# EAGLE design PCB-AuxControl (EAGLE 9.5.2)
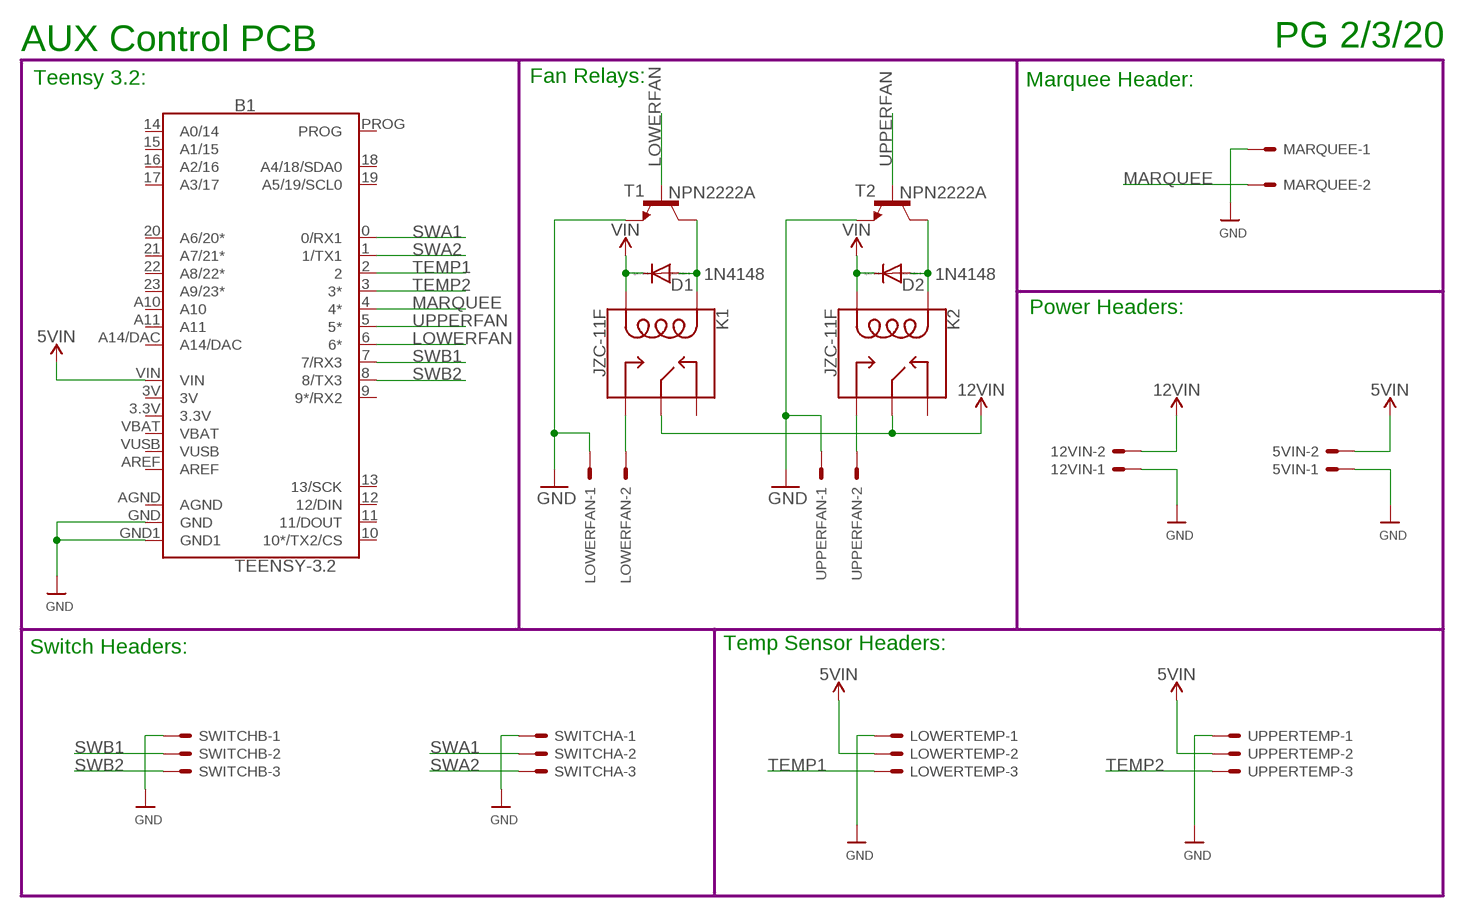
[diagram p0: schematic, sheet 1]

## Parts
5VIN  KK-156-2  [KK-156-2]
12VIN  KK-156-2  [KK-156-2]
B1  TEENSY-3.2  TEENSY-3.1SILK  [TEENSY-3.1]
D1  1N4148  1N4148DO35-7  [DO35-7]
D2  1N4148  1N4148DO35-7  [DO35-7]
K1  JZC-11F  RELAY-SPDT-JZC-11F  [RELAY-JZC]
K2  JZC-11F  RELAY-SPDT-JZC-11F  [RELAY-JZC]
LOWERFAN  KK-156-2  [KK-156-2]
LOWERTEMP  KK-156-3  [KK-156-3]
MARQUEE  KK-156-2  [KK-156-2]
SWITCHA  KK-156-3  [KK-156-3]
SWITCHB  KK-156-3  [KK-156-3]
T1  NPN2222A  BC337  [TO92]
T2  NPN2222A  BC337  [TO92]
UPPERFAN  KK-156-2  [KK-156-2]
UPPERTEMP  KK-156-3  [KK-156-3]

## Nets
5VIN: 5VIN.2 B1.VIN D1.C D2.C K1.1(COIL2) K2.1(COIL2) LOWERTEMP.2 UPPERTEMP.2 ; supply symbol labelled VIN
12VIN: 12VIN.2 K1.4(MAIN) K2.4(MAIN)
GND: 5VIN.1 12VIN.1 B1.GND B1.GND1 LOWERFAN.1 LOWERTEMP.1 MARQUEE.1 SWITCHA.1 SWITCHB.1 T1.1(E) T2.1(E) UPPERFAN.1 UPPERTEMP.1
LOWERFAN: B1.6(6*) T1.2(B)
MARQUEE: B1.4(4*) MARQUEE.2
N$3: K2.3(NO) UPPERFAN.2
N$4: K1.3(NO) LOWERFAN.2
RELAY1: D1.A K1.5(COIL1) T1.3(C)
RELAY2: D2.A K2.5(COIL1) T2.3(C)
SWA1: B1.0(0/RX1) SWITCHA.2
SWA2: B1.1(1/TX1) SWITCHA.3
SWB1: B1.7(7/RX3) SWITCHB.2
SWB2: B1.8(8/TX3) SWITCHB.3
TEMP1: B1.2 LOWERTEMP.3
TEMP2: B1.3(3*) UPPERTEMP.3
UPPERFAN: B1.5(5*) T2.2(B)
Unconnected: B1.9(9*/RX2) B1.10(10*/TX2/CS) B1.11(11/DOUT) B1.12(12/DIN) B1.13(13/SCK) B1.14(A0/14) B1.15(A1/15) B1.16(A2/16) B1.17(A3/17) B1.18(A4/18/SDA0) B1.19(A5/19/SCL0) B1.20(A6/20*) B1.21(A7/21*) B1.22(A8/22*) B1.23(A9/23*) B1.A10 B1.A11 B1.A14/DAC B1.AREF B1.PROG K1.2(NC) K2.2(NC)

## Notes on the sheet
- AUX Control PCB | PG 2/3/20
- Teensy 3.2: | Fan Relays: | Marquee Header:
- Power Headers:
- Switch Headers: | Temp Sensor Headers:

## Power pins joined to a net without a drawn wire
3.3V: B1.3.3V
3V: B1.3V
AGND: B1.AGND
VBAT: B1.VBAT
VUSB: B1.VUSB

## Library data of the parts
5VIN 12VIN LOWERFAN MARQUEE UPPERFAN = con-molex:KK-156-2: KK 156 HEADER; MF: MOLEX; OC_FARNELL: unknown; OC_NEWARK: unknown
B1 = SparkFun-Boards:TEENSY-3.1: Teensy 3+ Footprint Mechanical footprint with connectors for Teensy Development Board with ARM Cortex. SparkFun Products: Teensy 3.2 Teensy LC; SF_ID: DEV-12646
D1 D2 = diode:1N4148: DIODE
K1 K2 = SparkFun-Electromechanical:RELAY-SPDT: SPDT Electromechanical Relay Single-pole, double-throw sealed relays. When current is applied to the coil, it throws a simple changeover switch, terminating the connection from the NC contact to ground and closing the NO contact. Use them to switch high voltage/high current devices. SparkFun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; PROD_ID: COMP-09533; SF_SKU: COM-00100
LOWERTEMP SWITCHA SWITCHB UPPERTEMP = con-molex:KK-156-3: KK 156 HEADER Source: http://www.molex.com/pdm_docs/sd/026604100_sd.pdf; MF: MOLEX; OC_FARNELL: unknown; OC_NEWARK: unknown
T1 T2 = transistor:BC337: NPN TRANSISTOR

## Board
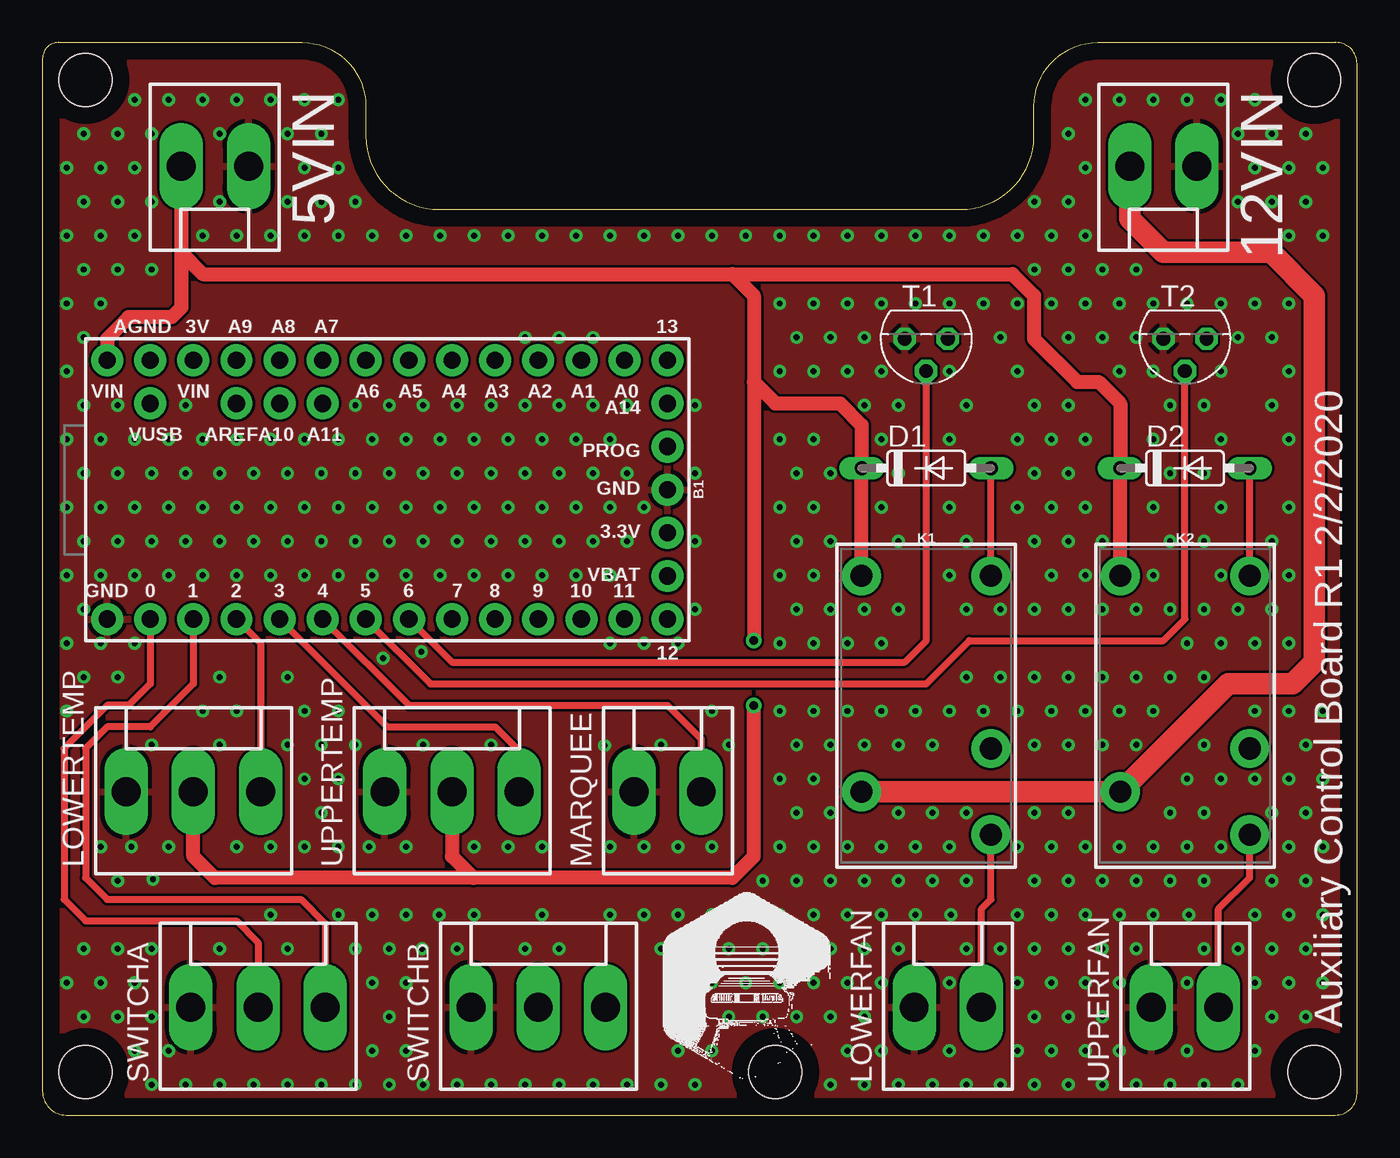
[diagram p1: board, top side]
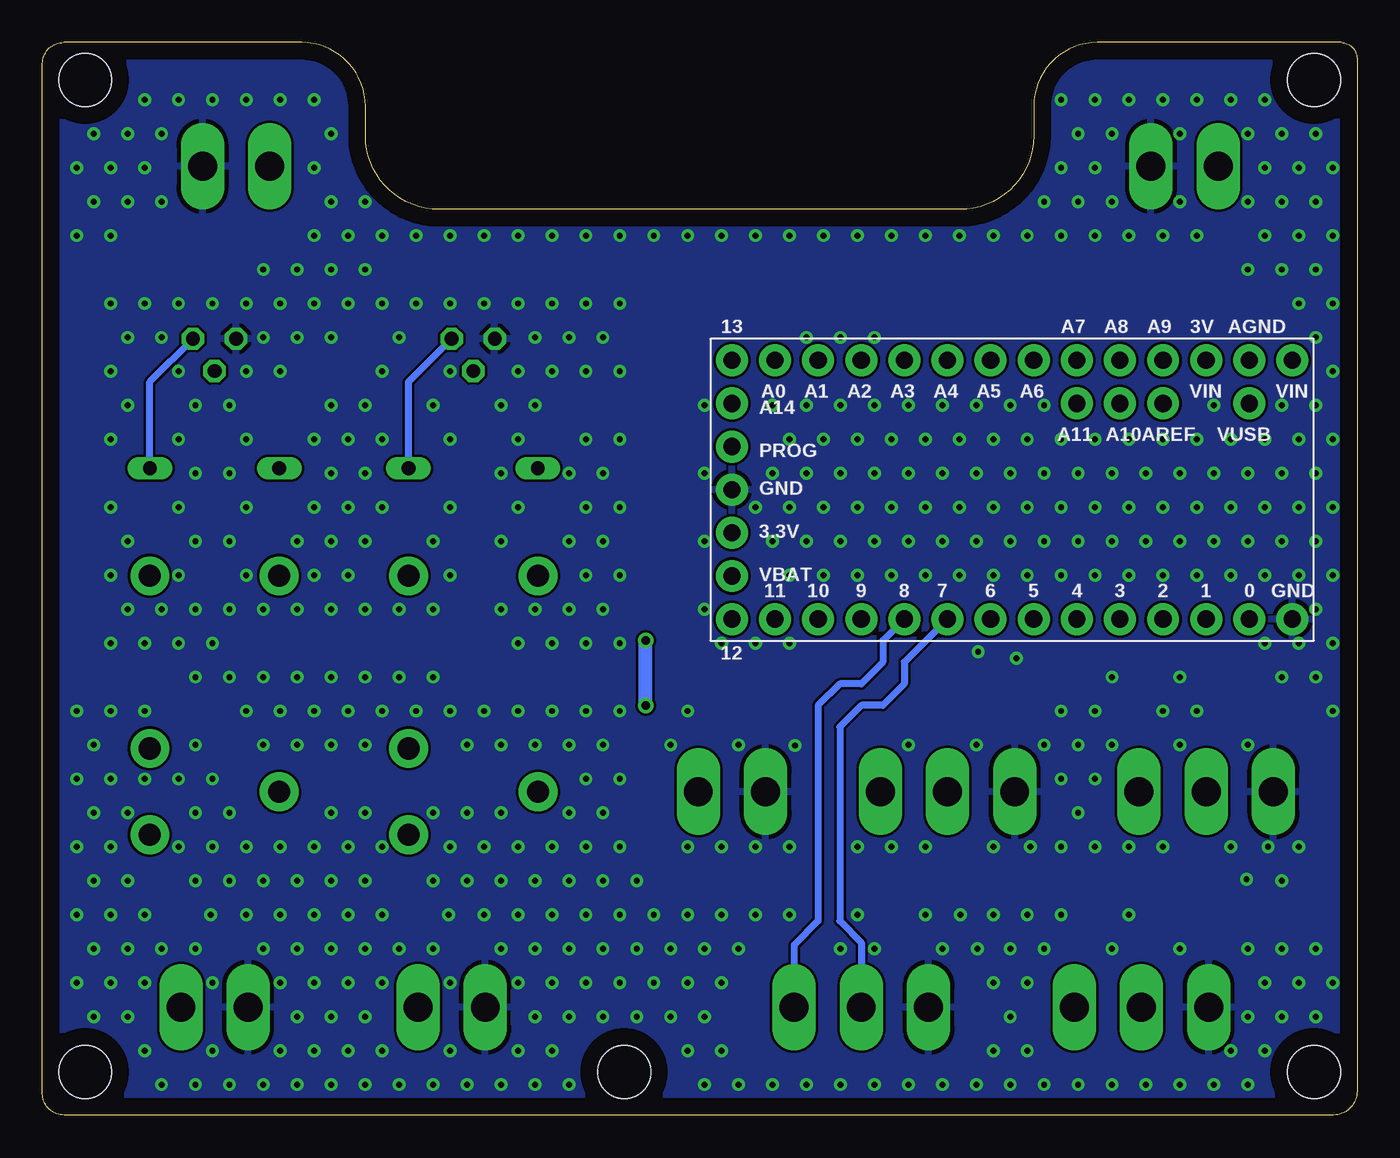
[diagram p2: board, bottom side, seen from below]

Size 77.45 x 63.17 mm. Coordinates in mm from the lower left corner, seen from the top.
Outline: 0,62.23 0,1.4 arc90 1.4,0 76.18,0 arc90 77.45,1.27 77.45,61.92 arc90 76.2,63.17 62.17,63.17 arc90 58.42,59.41 58.42,57.68 arc-90 54.08,53.34 23.39,53.34 arc-90 19.05,57.68 19.05,59.41 arc90 15.29,63.17 0.94,63.17 arc90 0,62.23
Copper layers (1*16): Top 0.035mm / dielectric 1.5mm / Bottom 0.035mm
Design rules "default": minimum track width 6mil, minimum drill 0.35mm, track to track 6mil, track to pad 6mil, pad to pad 6mil, via to via 6mil, smd to smd 6mil, copper to edge 40mil, drill to drill 6mil, minimum pad ring 10mil, minimum via ring 8mil, stop-mask expansion 4mil, vias tented up to drill 0.5mm, thermal gap 10mil
Holes 3.1 mm at 2.54,2.54 74.93,2.54 74.93,60.96 2.54,60.96 43.18,2.54

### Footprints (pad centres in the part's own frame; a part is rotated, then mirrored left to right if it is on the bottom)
KK-156-2 = drill 1.7 pad 2.184 long: 1 -1.98,0; 2 1.98,0
TEENSY-3.1 = drill 1.016 pad 1.88: 0 7.62,-13.97; 1 7.62,-11.43; 2 7.62,-8.89; 3 7.62,-6.35; 3.3V 2.54,16.51; 3V -7.62,-11.43; 4 7.62,-3.81; 5 7.62,-1.27; 6 7.62,1.27; 7 7.62,3.81; 8 7.62,6.35; 9 7.62,8.89; 10 7.62,11.43; 11 7.62,13.97; 12 7.62,16.51; 13 -7.62,16.51; 14 -7.62,13.97; 15 -7.62,11.43; 16 -7.62,8.89; 17 -7.62,6.35; 18 -7.62,3.81; 19 -7.62,1.27; 20 -7.62,-1.27; 21 -7.62,-3.81; 22 -7.62,-6.35; 23 -7.62,-8.89; A10 -5.08,-6.35; A11 -5.08,-3.81; A14/DAC -5.08,16.51; AGND -7.62,-13.97; AREF -5.08,-8.89; GND 0,16.51; GND1 7.62,-16.51; PROG -2.54,16.51; VBAT 5.08,16.51; VIN -7.62,-16.51; VUSB -5.08,-13.97
DO35-7 = drill 0.813 long: A 3.81,0; C -3.81,0
RELAY-JZC = drill 1.3 pad 2.286: 1 3.81,-8.89; 2 -3.81,1.27; 3 -3.81,6.35; 4 3.81,3.81; 5 -3.81,-8.89
KK-156-3 = drill 1.7 pad 2.184 long: 1 -3.96,0; 2 0,0; 3 3.96,0
TO92 = drill 0.813 octagon: 1 1.27,0; 2 0,1.905; 3 -1.27,0

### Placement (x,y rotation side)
5VIN  10.16,55.88 180 top
12VIN  66.04,55.88 180 top
B1  20.32,36.83 270 top
D1  52.07,38.1 0 top
D2  67.31,38.1 0 top
K1  52.07,22.86 180 top
K2  67.31,22.86 180 top
LOWERFAN  53.34,6.35 0 top
LOWERTEMP  8.89,19.05 0 top
MARQUEE  36.83,19.05 0 top
SWITCHA  12.7,6.35 0 top
SWITCHB  29.21,6.35 0 top
T1  52.07,45.72 180 top
T2  67.31,45.72 180 top
UPPERFAN  67.31,6.35 0 top
UPPERTEMP  24.13,19.05 0 top

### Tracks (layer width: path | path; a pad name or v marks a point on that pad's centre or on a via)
5VIN  (via drill 0.5)
  Top 0.813: K2.1 D2.C 63.5,41.91 62.23,43.18 60.96,43.18 58.42,45.72 58.42,48.26 57.15,49.53 40.64,49.53 | K1.1 D1.C 48.26,40.64 46.99,41.91 43.18,41.91 41.91,43.18 | 25.4,13.97 40.64,13.97 41.91,15.24 v41.91,24.13 | 25.4,13.97 10.16,13.97 8.89,15.24 LOWERTEMP.2 | 41.91,43.18 v41.91,27.94 | 40.64,49.53 41.91,48.26 41.91,43.18 | B1.VIN 3.81,45.72 5.08,46.99 7.62,46.99 8.18,47.55 8.18,50.8 | 5VIN.2 8.18,50.8 | 8.18,50.8 9.45,49.53 40.64,49.53 | UPPERTEMP.2 24.13,15.24 25.4,13.97
  Bottom 0.813: v41.91,24.13 v41.91,27.94
12VIN
  Top 1.27: K1.4 K2.4 69.85,25.4 73.66,25.4 74.93,26.67 74.93,48.26 72.39,50.8 66.04,50.8 64.06,52.78 12VIN.2
GND  (via drill 0.35)
  other vias: 2.44,5.8 1.44,7.8 2.44,9.8 1.44,23.8 2.44,25.8 1.44,27.8 2.44,29.8 1.44,31.8 2.44,33.8 1.44,35.8 2.44,37.8 1.44,39.8 2.44,41.8 1.44,43.8 2.44,45.8 1.44,47.8 2.44,49.8 1.44,51.8 2.44,53.8 1.44,55.8 2.44,57.8 4.44,5.8 3.44,7.8 4.44,9.8 4.44,13.8 3.44,15.8 4.44,25.8 3.44,27.8 3.44,31.8 4.44,33.8 3.44,35.8 4.44,37.8 3.44,39.8 4.44,41.8 3.44,47.8 4.44,49.8 3.44,51.8 4.44,53.8 3.44,55.8 4.44,57.8 6.44,1.8 5.44,3.8 6.44,5.8 5.44,7.8 6.44,9.8 6.44,21.8 5.44,27.8 5.44,31.8 6.44,33.8 5.44,35.8 6.44,37.8 5.44,39.8 6.44,49.8 5.44,51.8 6.44,53.8 5.44,55.8 6.44,57.8 5.44,59.8 8.44,1.8 7.44,3.8 7.44,15.8 7.44,31.8 8.44,33.8 7.44,35.8 8.44,37.8 7.44,39.8 8.44,41.8 7.44,59.8 10.44,1.8 10.44,9.8 5.24,15.8 10.44,21.8 9.44,23.8 10.44,25.8 9.44,31.8 10.44,33.8 9.44,35.8 10.44,37.8 9.44,39.8 9.44,51.8 10.44,53.8 10.44,57.8 9.44,59.8 12.44,1.8 11.44,15.8 11.44,23.8 11.44,31.8 12.44,33.8 11.44,35.8 12.44,37.8 11.44,39.8 11.44,51.8 11.44,59.8 14.44,1.8 14.44,9.8 13.44,11.8 13.44,15.8 14.44,21.8 14.44,25.8 13.44,31.8 14.44,33.8 13.44,35.8 14.44,37.8 13.44,39.8 13.44,51.8 14.44,53.8 14.44,57.8 13.44,59.8 16.44,1.8 15.44,15.8 16.44,17.8 15.44,19.8 16.44,21.8 15.44,23.8 15.44,31.8 16.44,33.8 15.44,35.8 16.44,37.8 15.44,39.8 15.44,51.8 16.44,53.8 15.44,55.8 16.44,57.8 15.44,59.8 18.44,1.8 18.44,9.8 17.44,11.8 17.44,15.8 17.44,19.8 18.44,21.8 17.44,23.8 17.44,31.8 18.44,33.8 17.44,35.8 18.44,37.8 17.44,39.8 18.44,41.8 17.44,51.8 18.44,53.8 17.44,55.8 17.44,59.8 20.44,1.8 19.44,3.8 20.44,5.8 19.44,7.8 20.44,9.8 19.44,11.8 20.07,26.91 19.44,31.8 20.44,33.8 19.44,35.8 20.44,37.8 19.44,39.8 20.44,41.8 19.44,51.8 22.44,1.8 21.44,3.8 21.44,7.8 21.44,11.8 21.44,15.8 22.44,21.8 22.32,27.29 21.44,31.8 22.44,33.8 21.44,35.8 22.44,37.8 21.44,39.8 22.44,41.8 21.44,51.8 24.44,1.8 24.44,9.8 19.24,15.8 23.44,31.8 24.44,33.8 23.44,35.8 24.44,37.8 23.44,39.8 24.44,41.8 23.44,51.8 26.44,1.8 6.51,13.89 22.37,9.8 25.44,11.8 25.44,15.8 26.44,21.8 25.44,31.8 26.44,33.8 25.44,35.8 26.44,37.8 25.44,39.8 26.44,41.8 25.44,51.8 28.44,1.8 28.44,9.8 23.37,11.8 27.44,15.8 27.44,31.8 28.44,33.8 27.44,35.8 28.44,37.8 27.44,39.8 28.44,41.8 28.44,45.8 27.44,51.8 30.44,1.8 30.44,9.8 29.44,11.8 29.44,15.8 29.44,31.8 30.44,33.8 29.44,35.8 30.44,37.8 29.44,39.8 30.44,41.8 30.44,45.8 29.44,51.8 32.44,1.8 31.44,31.8 32.44,33.8 31.44,35.8 32.44,37.8 31.44,39.8 32.44,41.8 32.44,45.8 31.44,51.8 34.44,1.8 33.44,11.8 33.44,15.8 33.44,27.8 33.44,31.8 34.44,33.8 33.44,35.8 34.44,37.8 33.44,39.8 34.44,41.8 33.44,51.8 36.44,1.8 36.44,9.8 35.44,11.8 35.44,15.8 36.44,21.8 35.44,27.8 35.44,35.8 35.44,51.8 38.44,1.8 37.44,3.8 38.44,5.8 37.44,7.8 38.44,9.8 37.44,11.8 37.44,15.8 33.12,21.76 37.44,27.8 38.44,29.8 38.44,33.8 38.44,37.8 38.44,41.8 37.44,51.8 39.44,3.8 40.44,5.8 39.44,7.8 40.44,9.8 39.44,11.8 39.44,15.8 40.44,21.8 39.44,23.8 39.44,51.8 42.44,5.8 41.44,7.8 42.44,9.8 41.44,11.8 42.44,13.8 41.44,51.8 44.44,5.8 43.44,7.8 44.44,9.8 43.44,11.8 44.44,13.8 43.44,15.8 44.44,17.8 43.44,19.8 44.44,21.8 43.44,23.8 43.44,27.8 44.44,29.8 43.44,31.8 44.44,33.8 43.44,35.8 44.44,37.8 43.44,39.8 43.44,43.8 44.44,45.8 43.44,47.8 43.44,51.8 46.44,1.8 46.44,5.8 45.44,7.8 46.44,9.8 45.44,11.8 46.44,13.8 45.44,15.8 46.44,17.8 45.44,19.8 46.44,21.8 45.44,23.8 45.44,27.8 46.44,29.8 45.44,31.8 46.44,33.8 45.44,35.8 46.44,37.8 45.44,39.8 45.44,43.8 46.44,45.8 45.44,47.8 45.44,51.8 48.44,1.8 47.44,3.8 48.44,5.8 47.44,7.8 48.44,9.8 47.44,11.8 48.44,13.8 47.44,15.8 48.44,21.8 47.44,23.8 47.44,27.8 48.44,29.8 48.44,41.8 47.44,43.8 48.44,45.8 47.44,47.8 47.44,51.8 50.44,1.8 49.44,3.8 49.44,7.8 50.44,9.8 49.44,11.8 50.44,13.8 49.44,15.8 50.44,17.8 50.44,21.8 49.44,23.8 49.44,27.8 50.44,29.8 50.44,33.8 49.44,35.8 50.44,37.8 49.44,39.8 50.44,41.8 49.44,43.8 49.44,47.8 49.44,51.8 52.44,1.8 51.44,11.8 52.44,13.8 51.44,15.8 52.44,17.8 52.44,21.8 51.44,23.8 51.44,47.8 51.44,51.8 54.44,1.8 53.44,3.8 53.44,7.8 54.44,9.8 54.44,13.8 53.44,15.8 54.44,17.8 53.44,23.8 54.44,25.8 54.44,29.8 53.44,31.8 54.44,33.8 53.44,35.8 53.44,39.8 54.44,41.8 53.44,43.8 53.44,47.8 53.44,51.8 56.44,1.8 56.44,9.8 53.53,11.8 55.44,23.8 56.44,25.8 56.44,29.8 56.44,45.8 55.44,47.8 55.44,51.8 58.44,1.8 57.44,3.8 58.44,5.8 57.44,7.8 58.44,9.8 57.44,11.8 58.44,13.8 57.44,15.8 58.44,17.8 58.44,21.8 57.44,23.8 58.44,25.8 58.44,29.8 58.44,33.8 57.44,35.8 58.44,37.8 57.44,39.8 58.44,41.8 57.44,43.8 57.44,47.8 58.44,49.8 57.44,51.8 58.44,53.8 60.44,1.8 59.44,3.8 60.44,5.8 59.44,7.8 60.44,9.8 59.44,11.8 60.44,13.8 59.44,15.8 60.44,17.8 60.44,21.8 59.44,23.8 60.44,25.8 60.44,29.8 59.44,31.8 60.44,33.8 59.44,35.8 60.44,37.8 59.44,39.8 60.44,41.8 60.44,45.8 59.44,47.8 60.44,49.8 59.44,51.8 60.44,53.8 60.44,57.8 62.44,1.8 61.44,3.8 62.44,5.8 61.44,7.8 62.44,9.8 61.44,11.8 62.44,13.8 61.44,15.8 62.44,21.8 61.44,23.8 62.44,25.8 62.44,29.8 61.44,31.8 62.44,33.8 61.44,35.8 61.44,39.8 62.44,45.8 61.44,47.8 62.44,49.8 61.44,51.8 61.44,55.8 61.44,59.8 64.44,1.8 63.44,3.8 63.44,7.8 64.44,9.8 63.44,11.8 64.44,13.8 63.44,15.8 64.44,21.8 63.44,23.8 64.44,25.8 64.44,29.8 63.44,43.8 64.44,45.8 63.44,47.8 64.44,49.8 63.44,59.8 66.44,1.8 65.44,11.8 66.44,13.8 65.44,15.8 66.44,17.8 65.44,23.8 66.44,25.8 66.44,29.8 65.44,31.8 66.44,33.8 65.44,35.8 66.44,37.8 65.44,39.8 66.44,41.8 65.44,43.8 65.44,47.8 65.44,59.8 68.44,1.8 67.44,3.8 67.44,7.8 68.44,9.8 68.44,13.8 67.44,15.8 68.44,17.8 67.44,19.8 68.44,21.8 68.44,25.8 67.44,27.8 68.44,29.8 68.44,33.8 68.44,37.8 68.44,41.8 67.44,47.8 67.44,59.8 70.44,1.8 70.44,9.8 67.53,11.8 69.44,15.8 69.44,19.8 69.44,27.8 70.44,29.8 69.44,31.8 69.44,35.8 69.44,39.8 69.44,43.8 70.44,45.8 69.44,47.8 70.44,53.8 70.44,57.8 69.44,59.8 71.44,3.8 72.44,5.8 71.44,7.8 72.44,9.8 71.44,11.8 72.44,13.8 72.44,17.8 71.44,19.8 71.44,23.8 71.44,27.8 72.44,29.8 72.44,33.8 72.44,41.8 72.44,45.8 71.44,47.8 72.44,53.8 71.44,55.8 72.44,57.8 71.44,59.8 74.44,5.8 73.44,7.8 74.44,9.8 73.44,11.8 74.44,13.8 73.44,15.8 74.44,17.8 73.44,19.8 74.44,21.8 73.44,23.8 73.44,27.8 73.44,31.8 73.44,35.8 73.44,39.8 73.44,43.8 73.44,47.8 73.44,51.8 74.44,53.8 73.44,55.8 74.44,57.8 75.44,7.8 75.44,11.8 75.44,15.8 75.44,19.8 75.44,23.8 75.44,51.8 75.44,55.8
  pour Top: 0,0 0,63.5 77.47,63.5 77.47,0
  pour Bottom: 0,0 0,63.5 77.47,63.5 77.47,0
LOWERFAN
  Top 0.406: B1.6 24.13,26.67 50.8,26.67 52.07,27.94 T1.2
MARQUEE
  Top 0.406: B1.4 21.59,24.13 36.83,24.13 38.81,22.15 MARQUEE.2
N$3
  Top 0.406: UPPERFAN.2 69.29,12.14 71.12,13.97 K2.3
N$4
  Top 0.406: LOWERFAN.2 55.32,12.14 55.88,12.7 K1.3
RELAY1
  Top 0.406: K1.5 D1.A
  Bottom 0.406: D1.A 55.88,43.18 T1.3
RELAY2
  Top 0.406: K2.5 D2.A
  Bottom 0.406: D2.A 71.12,43.18 T2.3
SWA1
  Top 0.406: B1.0 6.35,25.4 5.08,24.13 3.81,24.13 1.27,21.59 1.27,12.7 2.54,11.43 11.43,11.43 12.7,10.16 SWITCHA.2
SWA2
  Top 0.406: B1.1 8.89,25.4 6.35,22.86 3.81,22.86 2.54,21.59 2.54,13.97 3.81,12.7 15.24,12.7 16.66,11.28 SWITCHA.3
SWB1
  Bottom 0.406: B1.7 26.67,26.67 26.67,25.4 27.94,24.13 29.21,24.13 30.48,22.86 30.48,11.43 29.21,10.16 SWITCHB.2
SWB2
  Bottom 0.406: B1.8 27.94,27.94 27.94,26.67 29.21,25.4 30.48,25.4 31.75,24.13 31.75,11.43 33.17,10.01 SWITCHB.3
TEMP1
  Top 0.406: B1.2 12.85,27.79 LOWERTEMP.3
TEMP2
  Top 0.406: B1.3 20.32,22.86 26.67,22.86 27.94,21.59 27.94,20.47 28.09,20.32 UPPERTEMP.3
UPPERFAN
  Top 0.406: B1.5 22.86,25.4 52.07,25.4 54.61,27.94 66.04,27.94 67.31,29.21 T2.2

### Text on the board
tNames: Auxiliary Control Board R1 2/2/2020

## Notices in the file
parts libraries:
SparkFun-Electromechanical: Licensing: Creative Commons ShareAlike 4.0 International - https://creativecommons.org/licenses/by-sa/4.0
